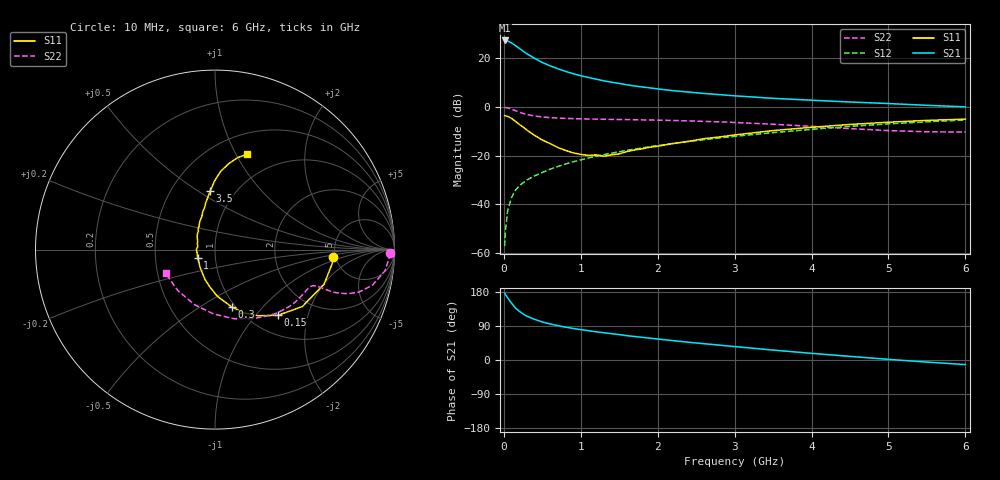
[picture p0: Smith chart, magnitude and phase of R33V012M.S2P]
! SIEMENS Small Signal Semiconductors
! BFR181
! Si NPN RF Bipolar Junction Transistor in SOT23
! VCE = 3 V  IC = 12 mA
! Common Emitter S-Parameters:  May  1996
# GHz  S  MA  R  50
!  f  S11  S21  S12  S22
! GHz  MAG  ANG  MAG  ANG  MAG  ANG  MAG  ANG
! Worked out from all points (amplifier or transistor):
!   36 points, 10 MHz to 6 GHz, reference 50 ohm
!   highest |S21| = 27.2 dB at 10 MHz (marker M1)
!   |S21| within 3 dB of that: start of sweep to 190.4 MHz
!   unconditionally stable (mu >= 1): 654.1 MHz to 2.594 GHz
!   at 250 MHz: K = 0.68, MSG = 27.0 dB, |S12| = -31.1 dB
!   at 1.4 GHz: K = 1.07, MAG = 12.9 dB, |S12| = -19.0 dB
!   at 6 GHz: K = 0.86, MSG = 2.7 dB, |S12| = -5.4 dB
!   S11 on the Smith chart (normalised r, x): 10 MHz: 4.80, -0.71; 150 MHz: 1.34, -1.32; 300 MHz: 0.96, -0.70; 1 GHz: 0.82, -0.07; 3.5 GHz: 0.77, +0.56; 6 GHz: 0.72, +1.11
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0.01  0.6613 -3.6  22.96 176.5  0.0014 97.5  0.9775 -1.2
0.02  0.6571 -7.0  22.67 173.1  0.0029 79.0  0.9707 -2.8
0.05  0.6376 -17.6  22.36 163.9  0.0075 81.5  0.9557 -7.0
0.1  0.5808 -33.1  20.44 150.0  0.0139 76.4  0.9 -12.7
0.15  0.5072 -46.2  18.03 137.6  0.0195 72.3  0.8375 -16.4
0.2  0.4398 -56.9  15.86 128.6  0.0242 70.1  0.7796 -18.4
0.25  0.3861 -65.7  13.87 121.4  0.0278 68.5  0.7338 -19.3
0.3  0.3345 -73.5  12.26 115.6  0.0319 69.1  0.7002 -19.8
0.4  0.2608 -87.0  9.857 107.2  0.0386 69.4  0.6512 -19.8
0.5  0.2093 -98.1  8.123 100.3  0.0453 69.7  0.6214 -19.7
0.6  0.1772 -107.9  6.959 95.2  0.0528 70.5  0.6026 -19.7
0.7  0.1474 -118.9  6.065 90.7  0.0599 71.1  0.5893 -20.0
0.8  0.1285 -130.9  5.345 86.8  0.0673 71.1  0.5816 -20.2
1  0.1063 -155.5  4.355 80.1  0.0819 71.5  0.5689 -21.5
1.1  0.1016 -167.1  4.006 77.4  0.0898 71.3  0.5647 -22.3
1.3  0.0974 171.6  3.419 71.9  0.1051 71.0  0.557 -24.1
1.6  0.1216 144.6  2.832 64.2  0.1286 69.8  0.5482 -27.5
2.2  0.1775 118.7  2.149 51.1  0.1781 66.7  0.5265 -35.8
3.5  0.3269 94.7  1.497 26.2  0.2967 55.9  0.4411 -60.6
4.5  0.4366 85.9  1.259 9.5  0.3984 44.6  0.3586 -91.4
5.5  0.529 76.0  1.076 -5.5  0.4952 31.1  0.3084 -132.1
6  0.5607 71.3  1.002 -12.1  0.5386 23.8  0.3059 -154.3
